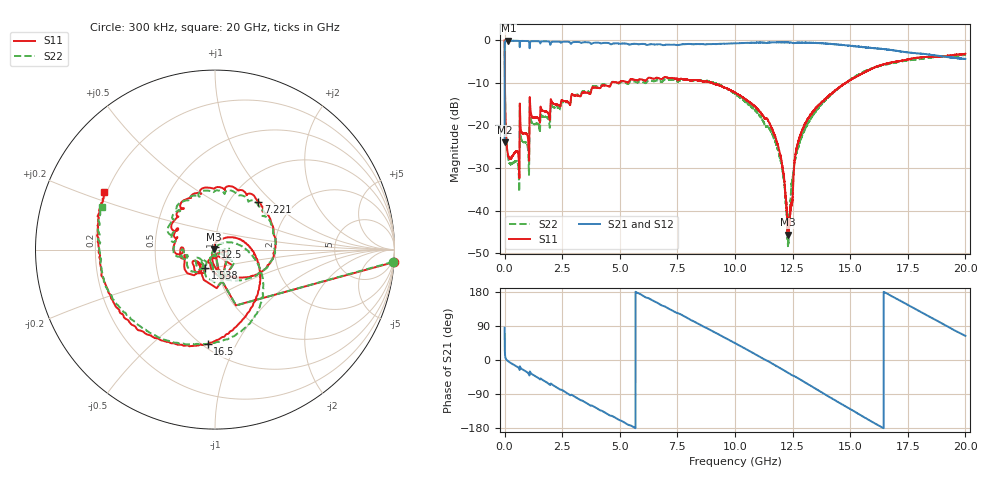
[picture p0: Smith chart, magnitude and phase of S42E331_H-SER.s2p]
! Created Wed Nov 25 22:12:26 2020
# khz S ma R 50
! 2 Port Network Data from SP1.SP block
! freq  magS11  angS11  magS21  angS21  magS12  angS12  magS22  angS22
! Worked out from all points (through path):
!   20001 points, 300 kHz to 20 GHz, reference 50 ohm
!   highest |S21| = -0.09 dB at 162.3 MHz (marker M1); lowest = -24.0 dB at 300 kHz (marker M2)
!   group delay of S21, straight-line fit = 91.6 ps
!   lowest |S11| = -45.7 dB at 12.3 GHz (marker M3), VSWR 1.01, Z = 49.5 + j0.153 ohm
!   |S11| at or under -10 dB: 14.05 MHz to 4.641 GHz (4.627 GHz wide, 199 % of centre); 9.006 GHz to 14.79 GHz (5.788 GHz wide, 48.6 % of centre); 14.79437 GHz to 14.8072 GHz (12.83 MHz wide, 0.0867 % of centre)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
!   |S22| runs from -48.4 to 0.0 dB; largest |S21 - S12| = 0.019
!   S11 on the Smith chart (normalised r, x): 300 kHz: 1, -28; 1.538 GHz: 0.88, -0.18; 7.221 GHz: 1.35, +0.83; 12.5 GHz: 1.00, +0.03; 16.5 GHz: 0.53, -0.78; 20 GHz: 0.19, +0.24
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300  0.9972 -4.1  0.06342 85.3  0.06366 85.8  0.9948 -3.9
162300  0.04366 -81.7  0.9896 -3.8  0.9884 -3.8  0.0404 -80.6
545300  0.04977 -99.3  0.988 -17.9  0.9867 -17.9  0.03752 -95.9
747300  0.08225 -110.0  0.9845 -23.6  0.984 -23.6  0.06622 -108.3
1538300  0.1151 -117.9  0.9365 -51.3  0.9365 -51.3  0.08791 -119.3
3334300  0.2329 163.5  0.9351 -106.5  0.9337 -106.6  0.2397 169.8
5198300  0.33 106.6  0.919 -164.9  0.9197 -165.0  0.3198 109.5
6667300  0.3611 62.4  0.9002 149.6  0.899 149.5  0.3374 59.1
7221300  0.3606 47.8  0.8873 132.3  0.8871 132.3  0.3435 40.8
8547300  0.3325 -0.7  0.9046 91.1  0.9039 91.1  0.3377 3.5
1.00003e7  0.2445 -38.6  0.923 44.5  0.924 44.6  0.2362 -45.3
1.16583e7  0.0842 -94.5  0.9479 -11.0  0.9486 -11.0  0.07402 -109.9
1.20373e7  0.03603 -117.7  0.9505 -24.2  0.949 -24.3  0.03222 -126.7
1.22973e7  0.005186 162.7  0.9468 -33.6  0.9503 -33.6  0.003915 157.0
1.24983e7  0.01429 89.1  0.9327 -40.7  0.9328 -41.0  0.02327 59.8
1.27283e7  0.06155 62.2  0.9379 -48.1  0.94 -48.3  0.05477 42.2
1.33343e7  0.1383 26.6  0.9316 -69.9  0.9316 -69.7  0.126 14.9
1.51573e7  0.3626 -51.5  0.8508 -135.0  0.86 -135.3  0.3671 -43.1
1.64973e7  0.529 -94.4  0.7868 178.5  0.7744 178.7  0.5151 -89.0
1.66673e7  0.5365 -98.9  0.7786 173.3  0.763 173.0  0.5278 -95.2
1.83093e7  0.6371 -154.3  0.6864 118.5  0.6851 119.2  0.6181 -147.4
2e7  0.6969 152.3  0.6028 63.6  0.6035 64.6  0.676 159.3
